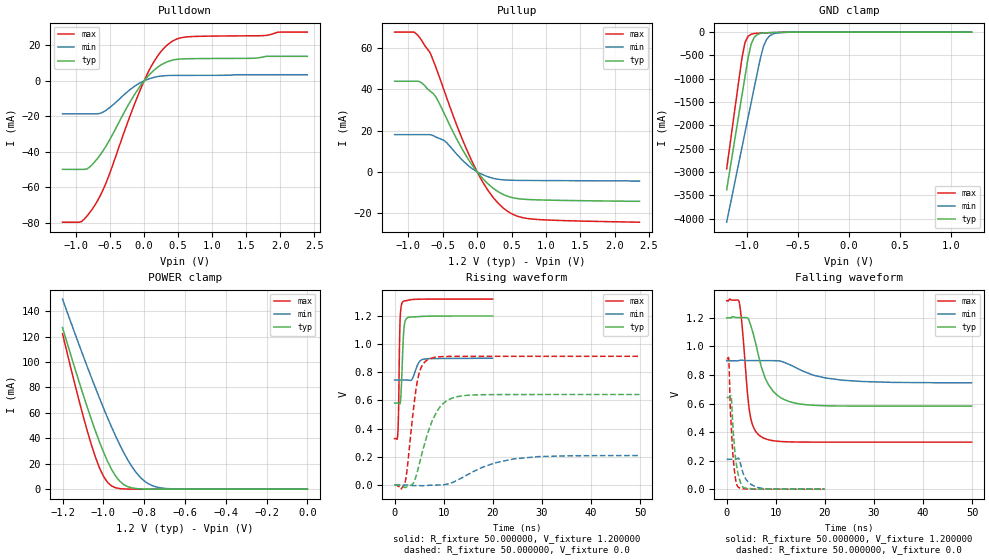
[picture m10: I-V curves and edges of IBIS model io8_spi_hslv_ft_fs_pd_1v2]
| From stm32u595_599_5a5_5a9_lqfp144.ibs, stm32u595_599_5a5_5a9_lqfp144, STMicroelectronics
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|   Model io8_spi_hslv_ft_fs_pd_1v2
[Model]  io8_spi_hslv_ft_fs_pd_1v2
Model_type I/O
Polarity   Non-Inverting
Enable   Active-Low
Vinl =   0.360000V
Vinh =   0.840000V
Vmeas =  0.600000V
Cref =   50.000000pF
Rref =   100.000000M
Vref =   0.0V
C_comp   3.133100pF   3.070300pF   3.178200pF
[Temperature Range]   25.000000   0.140000k   -40.000000
[Pullup Reference]   1.200000V   0.900000V   1.320000V
[Pulldown Reference]   0.0V   0.0V   0.0V
[POWER Clamp Reference]   1.200000V   0.900000V   1.320000V
[GND Clamp Reference]   0.0V   0.0V   0.0V
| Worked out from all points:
|   slope of the pulldown table from 0 to 0.18 V, typ, clamps not added: 25.4 ohm
|   slope of the pullup table from 0 to 0.18 V, typ, clamps not added: 27.8 ohm
|   GND clamp passes 1 mA (typ) near -0.51 V on its own axis
|   POWER clamp passes 1 mA (typ) near -0.86 V on its own axis
|   rising waveform, R_fixture 50.000000, V_fixture 1.200000: 20-80 % time 445ps typ, 1.04ns min, 266ps max; typ from 0.581 V to 1.2 V
|   rising waveform, R_fixture 50.000000, V_fixture 0.0: 20-80 % time 3.6ns typ, 8.6ns min, 1.83ns max; typ from 0 V to 0.642 V
|   falling waveform, R_fixture 50.000000, V_fixture 1.200000: 20-80 % time 3.56ns typ, 7.7ns min, 1.53ns max; typ from 1.2 V to 0.581 V
|   falling waveform, R_fixture 50.000000, V_fixture 0.0: 20-80 % time 1.04ns typ, 1.77ns min, 822ps max; typ from 0.642 V to 0 V
[Pulldown]
|Voltage   I(typ)   I(min)   I(max)
-1.2V     -49.85mA   -18.57mA   -79.56mA
-920mV    -49.85mA   -18.57mA   -79.19mA
-840mV    -49.59mA   -18.57mA   -76.08mA
-720mV    -45.32mA   -18.57mA   -69.74mA
-560mV    -36.71mA   -16.58mA   -57.44mA
-200mV    -11.43mA   -4.74mA    -19.03mA
0V        -10fA      -500fA     0A
160mV     6.476mA    2.075mA    11.78mA
360mV     10.99mA    2.989mA    20.81mA
480mV     12.07mA    3.053mA    23.52mA
640mV     12.42mA    3.074mA    24.76mA
2.4V      13.78mA    3.432mA    27.43mA
[Pullup]
|Voltage   I(typ)   I(min)   I(max)
-1.2V     43.98mA    18.03mA    67.82mA
-920mV    43.98mA    18.03mA    67.82mA
-840mV    43.85mA    18.03mA    65.38mA
-680mV    39.07mA    18.03mA    57.58mA
-600mV    36.37mA    16.87mA    50.73mA
-480mV    28.4mA     15.19mA    39.49mA
-280mV    14.84mA    7.942mA    21.22mA
-80mV     3.667mA    1.75mA     5.47mA
160mV     -5.889mA   -2.43mA    -9.115mA
400mV     -11.31mA   -3.958mA   -18.11mA
800mV     -13.54mA   -4.214mA   -22.92mA
2.36V     -14.3mA    -4.5mA     -24.46mA
[GND_clamp]
|Voltage   I(typ)   I(min)   I(max)
-1.2V     -3.379A    -4.076A    -2.932A
-1.05V    -1.35A     -2.47A     -550.7mA
-1.02V    -947.8mA   -2.15A     -221.5mA
-990mV    -552.4mA   -1.829A    -88.45mA
-960mV    -255.3mA   -1.51A     -44.89mA
-930mV    -111.8mA   -1.191A    -30.69mA
-870mV    -28.36mA   -564.6mA   -21.36mA
-840mV    -18.66mA   -309.5mA   -18.51mA
-810mV    -14.08mA   -161.6mA   -15.94mA
-780mV    -11.38mA   -83.33mA   -13.55mA
-600mV    -3.019mA   -4.329mA   -3.104mA
1.2V      30.28uA    18.17uA    37.27uA
[POWER_clamp]
|Voltage   I(typ)   I(min)   I(max)
-1.2V     127mA      149.4mA    122.2mA
-1.12V    84.97mA    114mA      70.27mA
-1.06V    55.51mA    88.42mA    35.67mA
-1.02V    37.63mA    72.04mA    17.17mA
-1V       29.51mA    64.13mA    10.3mA
-960mV    15.69mA    48.99mA    2.571mA
-900mV    3.624mA    28.77mA    182.8uA
-840mV    490.7uA    13.24mA    11.35uA
-800mV    116.8uA    6.532mA    1.77uA
-740mV    13.2uA     1.723mA    109.1nA
-620mV    167.4nA    79.36uA    0A
0V        0A         17.87nA    0A
[Ramp]
| variable   typ   min   max
dV/dt_r  0.38524/3.59586n   0.12537/8.59280n   0.54787/1.82382n
dV/dt_f  0.37090/3.55686n   92.55000m/7.71128n  0.59417/1.52927n
R_load = 50.000000
[Rising Waveform]
R_fixture= 50.000000
V_fixture= 1.200000
V_fixture_min= 0.900000
V_fixture_max= 1.320000
|time   V(typ)   V(min)   V(max)
0s        581.4mV    745.2mV    329.3mV
680.7ps   581.3mV    745.2mV    382.2mV
800.8ps   579.8mV    745.2mV    512.9mV
1.001ns   573.8mV    745.2mV    1.002V
1.121ns   579.3mV    745.2mV    1.173V
1.602ns   901.5mV    745.2mV    1.298V
1.962ns   1.129V     745.3mV    1.306V
2.643ns   1.188V     744.6mV    1.31V
5.846ns   1.197V     892.4mV    1.319V
19.94ns   1.2V       899.5mV    1.319V
[Rising Waveform]
R_fixture= 50.000000
V_fixture= 0.0
V_fixture_min= 0.0
V_fixture_max= 0.0
|time   V(typ)   V(min)   V(max)
0s        -1.829uV   1.339uV    -19.27uV
2.102ns   -17.17mV   5.497uV    13.66mV
3.704ns   8.27mV     -3.896mV   496.9mV
4.605ns   91.28mV    -3.837mV   732.6mV
5.506ns   214.4mV    -4.818mV   841.3mV
6.907ns   384.1mV    -2.031mV   892.6mV
9.51ns    564.9mV    857.5uV    910.8mV
13.31ns   630.4mV    43.83mV    913.1mV
24.22ns   642.1mV    185.3mV    913.3mV
49.85ns   642.2mV    209.1mV    913.3mV
[Falling Waveform]
R_fixture= 50.000000
V_fixture= 1.200000
V_fixture_min= 0.900000
V_fixture_max= 1.320000
|time   V(typ)   V(min)   V(max)
0s        1.2V       899.5mV    1.319V
2.503ns   1.202V     901mV      1.316V
3.103ns   1.202V     903.2mV    1.157V
4.705ns   1.167V     900.6mV    532.8mV
5.606ns   1.062V     900.3mV    423mV
7.207ns   840.3mV    900.2mV    363.5mV
9.51ns    683.5mV    899.9mV    339.4mV
14.51ns   599mV      843.8mV    330.1mV
23.42ns   582.5mV    763.8mV    329.3mV
49.85ns   581.4mV    745.2mV    329.3mV
[Falling Waveform]
R_fixture= 50.000000
V_fixture= 0.0
V_fixture_min= 0.0
V_fixture_max= 0.0
|time   V(typ)   V(min)   V(max)
0s        642.2mV    209.1mV    913.3mV
440.4ps   642.1mV    209.1mV    898.9mV
720.7ps   648mV      209.2mV    580.2mV
920.9ps   649.5mV    209.2mV    447.9mV
1.201ns   480.4mV    209.2mV    277.2mV
1.522ns   317.6mV    208.9mV    147.5mV
2.242ns   120mV      215.9mV    18.32mV
3.323ns   14.27mV    113mV      3.122mV
5.966ns   1.612mV    16.58mV    399.8uV
19.94ns   -1.829uV   1.339uV    -19.27uV
